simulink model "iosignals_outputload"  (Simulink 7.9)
settings: Solver=ode23s  StartTime=0.0  StopTime=400  RelTol=1e-6
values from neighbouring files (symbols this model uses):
  design = []    [sword.m]
libraries: simulink x1, cstextras x1

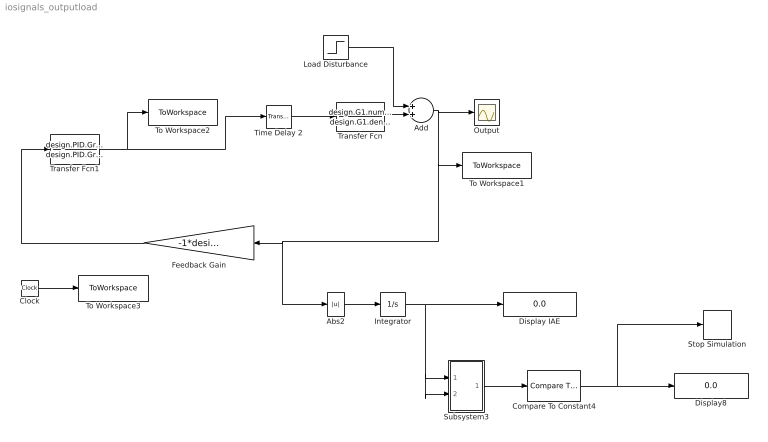
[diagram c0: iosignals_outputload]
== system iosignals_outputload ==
  Abs2 : Abs
  Add : Sum
  Clock : Clock
  Compare To Constant4 : simulink/Logic and Bit Operations/Compare To Constant  relop=<=  const=0.001  OutDataTypeStr=boolean  ZeroCross=off
  Display IAE : Display
  Display8 : Display
  Feedback Gain : Gain  Gain=-1*design.sim.sgn
  Integrator : Integrator
  Load Disturbance : Step  Time=0  SampleTime=0
  Output : Scope
  Stop Simulation : Stop
  Subsystem3 : Subsystem
  Time Delay 2 : cstextras/Transport Delay (masked)  Tag=InputDelayBlock  Td=design.sim.L1  u0=0  bufsize=100000
  To Workspace1 : ToWorkspace  VariableName=outputsignal  SampleTime=-1
  To Workspace2 : ToWorkspace  VariableName=controlsignal  SampleTime=-1
  To Workspace3 : ToWorkspace  VariableName=timesignal  SampleTime=-1
  Transfer Fcn : TransferFcn  Numerator=design.G1.num{1}  Denominator=design.G1.den{1}
  Transfer Fcn1 : TransferFcn  Numerator=design.PID.Grfinal.num{1}  Denominator=design.PID.Grfinal.den{1}
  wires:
  Transfer Fcn1/1 -> To Workspace2/1, Time Delay 2/1
  Feedback Gain/1 -> Transfer Fcn1/1
  Integrator/1 -> Display IAE/1, Subsystem3/2(In2), Subsystem3/1(In1)
  Subsystem3/1(Out1) -> Compare To Constant4/1
  Compare To Constant4/1 -> Display8/1, Stop Simulation/1
  Abs2/1 -> Integrator/1
  Clock/1 -> To Workspace3/1
  Time Delay 2/1 -> Transfer Fcn/1
  Transfer Fcn/1 -> Add/2
  Add/1 -> Output/1, To Workspace1/1, Feedback Gain/1, Abs2/1
  Load Disturbance/1 -> Add/1

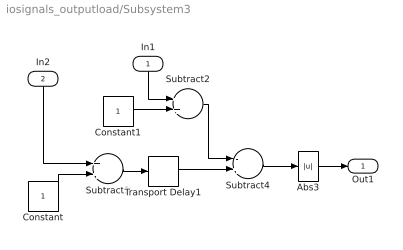
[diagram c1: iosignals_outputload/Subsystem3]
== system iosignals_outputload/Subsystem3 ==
  In1 : Inport
  In2 : Inport  Port=2
  Abs3 : Abs  ZeroCross=off
  Constant : Constant
  Constant1 : Constant
  Subtract1 : Sum
  Subtract2 : Sum
  Subtract4 : Sum  Inputs=-+
  Transport Delay1 : TransportDelay  DelayTime=50  BufferSize=10000
  Out1 : Outport
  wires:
  Abs3/1 -> Out1/1
  Subtract4/1 -> Abs3/1
  Transport Delay1/1 -> Subtract4/2
  Constant/1 -> Subtract1/2
  In2/1 -> Subtract1/1
  Subtract1/1 -> Transport Delay1/1
  Constant1/1 -> Subtract2/2
  Subtract2/1 -> Subtract4/1
  In1/1 -> Subtract2/1
